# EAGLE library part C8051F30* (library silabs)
25 MIPS, 8 kB Flash, 8-Bit ADC, 11-Pin Mixed-Signal MCU Source: http://www.silabs.com/products/microcontroller .. C8051F30xrev2_3.pdf
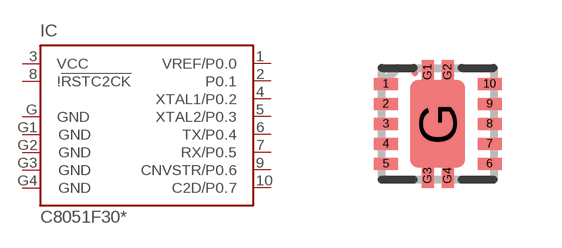
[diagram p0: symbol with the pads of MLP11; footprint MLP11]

Designator prefix IC

## C8051F300 (MPN: C8051F300-GM; OC_FARNELL: 4128310; OC_NEWARK: 96K8386), C8051F301 (MPN: C8051F301-GM; OC_FARNELL: 1291497; OC_NEWARK: 24M1228), C8051F302 (OC_FARNELL: 9685812; OC_NEWARK: unknown), C8051F303 (OC_FARNELL: unknown; OC_NEWARK: unknown), C8051F304 (MPN: C8051F304-GM; OC_FARNELL: 1291498; OC_NEWARK: 24M1229), C8051F305 (MPN: C8051F305-GM; OC_FARNELL: 1291499; OC_NEWARK: 24M1230)  [MLP11]
1  VREF/P0.0
2  P0.1
3  VCC  pwr
4  XTAL1/P0.2
5  XTAL2/P0.3
6  TX/P0.4
7  RX/P0.5
8  !!RSTC2CK  in
9  CNVSTR/P0.6
10  C2D/P0.7
G  GND  pwr
G1  GND  pwr
G2  GND  pwr
G3  GND  pwr
G4  GND  pwr

## Footprint MLP11 (pad centres in mm)
Tiny MLP package Source: http://www.silabs.com/products/microcontroller .. C8051F30xrev2_3.pdf
smd 0.6 x 0.3: 1 -1.3,1; 2 -1.3,0.5; 3 -1.3,0; 4 -1.3,-0.5; 5 -1.3,-1; 6 1.3,-1; 7 1.3,-0.5; 8 1.3,0; 9 1.3,0.5; 10 1.3,1
smd 1.36 x 2.2: G 0,0
smd 0.3 x 0.6: G1 -0.25,1.3; G2 0.25,1.3; G3 -0.25,-1.3; G4 0.25,-1.3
